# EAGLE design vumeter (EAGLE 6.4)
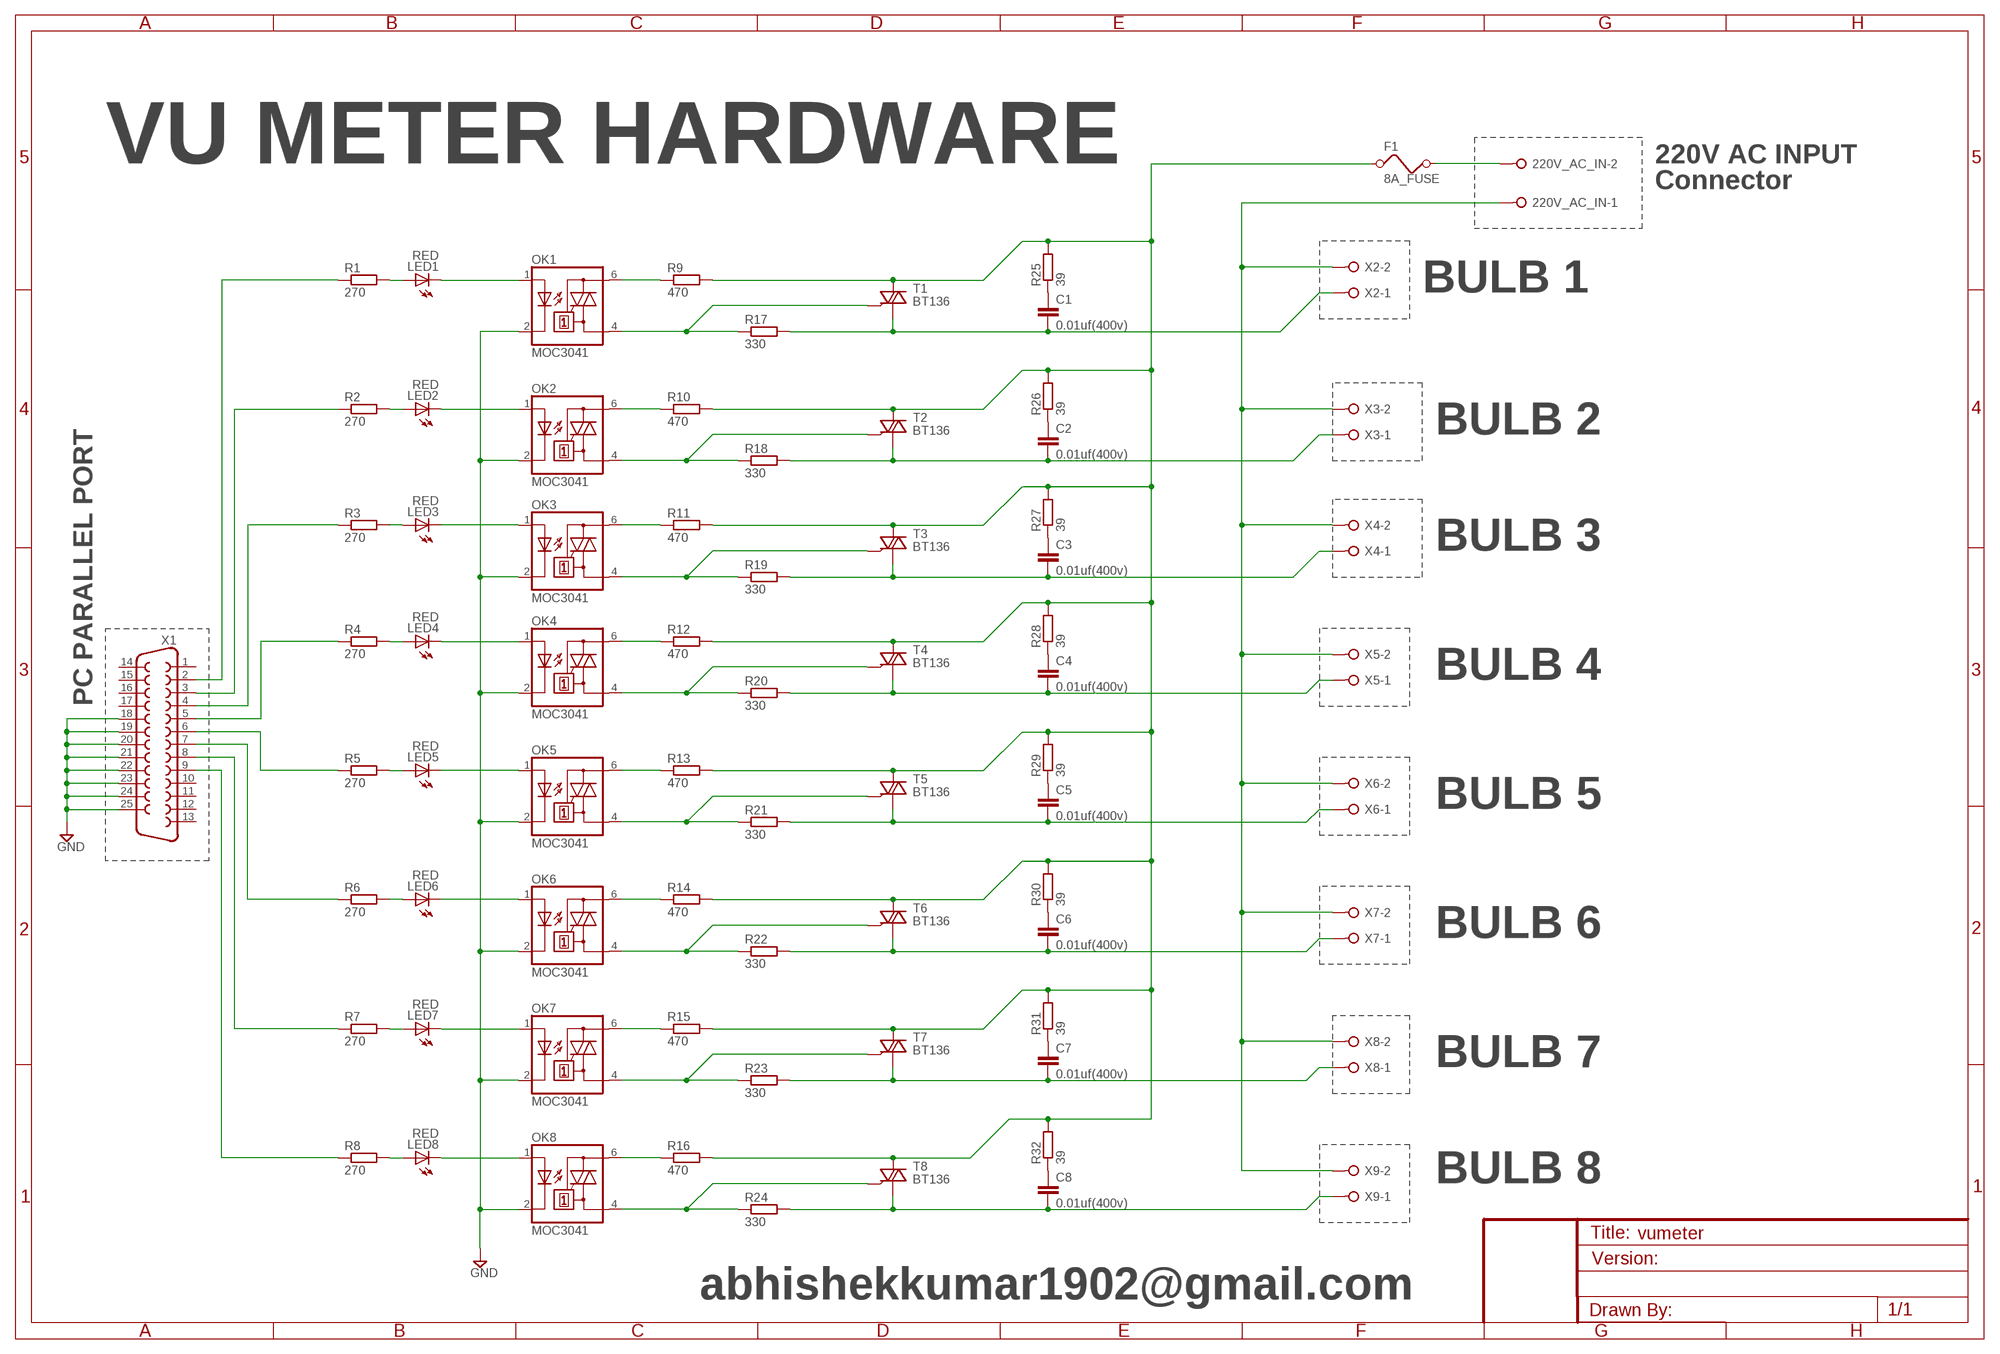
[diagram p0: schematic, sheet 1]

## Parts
220V_AC_IN  W237-02P  [W237-132]
C1  0.01uf(400v)  C-EU102-043X133  [C102-043X133]
C2  0.01uf(400v)  C-EU102-043X133  [C102-043X133]
C3  0.01uf(400v)  C-EU102-043X133  [C102-043X133]
C4  0.01uf(400v)  C-EU102-043X133  [C102-043X133]
C5  0.01uf(400v)  C-EU102-043X133  [C102-043X133]
C6  0.01uf(400v)  C-EU102-043X133  [C102-043X133]
C7  0.01uf(400v)  C-EU102-043X133  [C102-043X133]
C8  0.01uf(400v)  C-EU102-043X133  [C102-043X133]
F1  8A_FUSE  FUSE  [FUSE]
LED1  RED  LED3MM  [LED3MM]
LED2  RED  LED3MM  [LED3MM]
LED3  RED  LED3MM  [LED3MM]
LED4  RED  LED3MM  [LED3MM]
LED5  RED  LED3MM  [LED3MM]
LED6  RED  LED3MM  [LED3MM]
LED7  RED  LED3MM  [LED3MM]
LED8  RED  LED3MM  [LED3MM]
OK1  MOC3041  MOC3041T  [DIL06B]
OK2  MOC3041  MOC3041T  [DIL06B]
OK3  MOC3041  MOC3041T  [DIL06B]
OK4  MOC3041  MOC3041T  [DIL06B]
OK5  MOC3041  MOC3041T  [DIL06B]
OK6  MOC3041  MOC3041T  [DIL06B]
OK7  MOC3041  MOC3041T  [DIL06B]
OK8  MOC3041  MOC3041T  [DIL06B]
R1  270  R-EU_0309/12  [0309/12]
R2  270  R-EU_0309/12  [0309/12]
R3  270  R-EU_0309/12  [0309/12]
R4  270  R-EU_0309/12  [0309/12]
R5  270  R-EU_0309/12  [0309/12]
R6  270  R-EU_0309/12  [0309/12]
R7  270  R-EU_0309/12  [0309/12]
R8  270  R-EU_0309/12  [0309/12]
R9  470  R-EU_0309/12  [0309/12]
R10  470  R-EU_0309/12  [0309/12]
R11  470  R-EU_0309/12  [0309/12]
R12  470  R-EU_0309/12  [0309/12]
R13  470  R-EU_0309/12  [0309/12]
R14  470  R-EU_0309/12  [0309/12]
R15  470  R-EU_0309/12  [0309/12]
R16  470  R-EU_0309/12  [0309/12]
R17  330  R-EU_0309/12  [0309/12]
R18  330  R-EU_0309/12  [0309/12]
R19  330  R-EU_0309/12  [0309/12]
R20  330  R-EU_0309/12  [0309/12]
R21  330  R-EU_0309/12  [0309/12]
R22  330  R-EU_0309/12  [0309/12]
R23  330  R-EU_0309/12  [0309/12]
R24  330  R-EU_0309/12  [0309/12]
R25  39  R-EU_0309/12  [0309/12]
R26  39  R-EU_0309/12  [0309/12]
R27  39  R-EU_0309/12  [0309/12]
R28  39  R-EU_0309/12  [0309/12]
R29  39  R-EU_0309/12  [0309/12]
R30  39  R-EU_0309/12  [0309/12]
R31  39  R-EU_0309/12  [0309/12]
R32  39  R-EU_0309/12  [0309/12]
T1  BT136  [TO220AB]
T2  BT136  [TO220AB]
T3  BT136  [TO220AB]
T4  BT136  [TO220AB]
T5  BT136  [TO220AB]
T6  BT136  [TO220AB]
T7  BT136  [TO220AB]
T8  BT136  [TO220AB]
X1  F25HP  [F25HP]
X2  W237-02P  [W237-132]
X3  W237-02P  [W237-132]
X4  W237-02P  [W237-132]
X5  W237-02P  [W237-132]
X6  W237-02P  [W237-132]
X7  W237-02P  [W237-132]
X8  W237-02P  [W237-132]
X9  W237-02P  [W237-132]

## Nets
GND: OK1.2(C) OK2.2(C) OK3.2(C) OK4.2(C) OK5.2(C) OK6.2(C) OK7.2(C) OK8.2(C) X1.18 X1.19 X1.20 X1.21 X1.22 X1.23 X1.24 X1.25
N$1: LED5.A R5.2
N$2: LED1.A R1.2
N$3: LED1.K(C) OK1.1(A)
N$4: LED2.A R2.2
N$5: LED2.K(C) OK2.1(A)
N$6: LED3.K(C) OK3.1(A)
N$7: LED3.A R3.2
N$8: LED4.K(C) OK4.1(A)
N$9: LED4.A R4.2
N$10: LED6.A R6.2
N$11: LED7.A R7.2
N$12: LED8.A R8.2
N$13: LED8.K(C) OK8.1(A)
N$14: LED7.K(C) OK7.1(A)
N$15: LED6.K(C) OK6.1(A)
N$16: LED5.K(C) OK5.1(A)
N$17: R1.1 X1.2
N$18: R2.1 X1.3
N$19: R3.1 X1.4
N$20: R4.1 X1.5
N$21: R5.1 X1.6
N$22: R6.1 X1.7
N$23: R7.1 X1.8
N$24: R8.1 X1.9
N$25: 220V_AC_IN.1 X2.2 X3.2 X4.2 X5.2 X6.2 X7.2 X8.2 X9.2
N$26: OK5.6(A2) R13.1
N$27: OK6.6(A2) R14.1
N$28: OK7.6(A2) R15.1
N$29: OK8.6(A2) R16.1
N$30: OK4.6(A2) R12.1
N$31: OK3.6(A2) R11.1
N$32: OK2.6(A2) R10.1
N$33: OK1.6(A2) R9.1
N$34: OK1.4(A1) R17.1 T1.3(G)
N$35: OK2.4(A1) R18.1 T2.3(G)
N$36: OK3.4(A1) R19.1 T3.3(G)
N$37: OK4.4(A1) R20.1 T4.3(G)
N$38: OK5.4(A1) R21.1 T5.3(G)
N$39: OK6.4(A1) R22.1 T6.3(G)
N$40: OK7.4(A1) R23.1 T7.3(G)
N$41: OK8.4(A1) R24.1 T8.3(G)
N$42: C1.1 R25.1
N$43: C2.1 R26.1
N$44: C3.1 R27.1
N$45: C4.1 R28.1
N$46: C5.1 R29.1
N$47: C6.1 R30.1
N$48: C7.1 R31.1
N$49: C8.1 R32.1
N$50: F1.1 R9.2 R10.2 R11.2 R12.2 R13.2 R14.2 R15.2 R16.2 R25.2 R26.2 R27.2 R28.2 R29.2 R30.2 R31.2 R32.2 T1.2(A2) T2.2(A2) T3.2(A2) T4.2(A2) T5.2(A2) T6.2(A2) T7.2(A2) T8.2(A2)
N$51: C1.2 R17.2 T1.1(A1) X2.1
N$52: C7.2 R23.2 T7.1(A1) X8.1
N$59: C2.2 R18.2 T2.1(A1) X3.1
N$60: C3.2 R19.2 T3.1(A1) X4.1
N$61: C6.2 R22.2 T6.1(A1) X7.1
N$62: C5.2 R21.2 T5.1(A1) X6.1
N$63: C4.2 R20.2 T4.1(A1) X5.1
N$65: C8.2 R24.2 T8.1(A1) X9.1
N$66: 220V_AC_IN.2 F1.2
Unconnected: X1.1 X1.10 X1.11 X1.12 X1.13 X1.14 X1.15 X1.16 X1.17

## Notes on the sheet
- VU METER HARDWARE | 220V AC INPUT
- Connector
- BULB 1
- BULB 2
- BULB 3
- BULB 4
- PC PARALLEL PORT
- BULB 5
- BULB 6
- BULB 7
- BULB 8
- abhishekkumar1902@gmail.com

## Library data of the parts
220V_AC_IN X2-X9 = con-wago-508:W237-02P: WAGO SREW CLAMP; OC_FARNELL: unknown; OC_NEWARK: unknown
C1-C8 = resistor:C-EU: CAPACITOR, European symbol
F1 = special:FUSE: FUSE
LED1-LED8 = led:LED: LED
OK1-OK8 = optocoupler:MOC30*: 6-Pin DIP Zero-Cross Optoisolators Triac Driver Output (250/400 Volt Peak) Source: http://www.fairchildsemi.com/ds/MO/MOC3043-M.pdf; OC_FARNELL: unknown; OC_NEWARK: unknown
R1-R32 = resistor:R-EU_: RESISTOR, European symbol
T1-T8 = triac:BT136: Triac BT136 series E sensitive gate Source: http://www.nxp.com/acrobat_download/datasheets/BT136_SERIES_E_2.pdf
X1 = SparkFun:F25: D-SUB 25 25 Pin male connector. PCB edge mount for regular PCB thicknesses. This connector will connect directly to the back of a PC parallel port or through a normal DB25 extension cable (M/F). SKU: PRT-08287

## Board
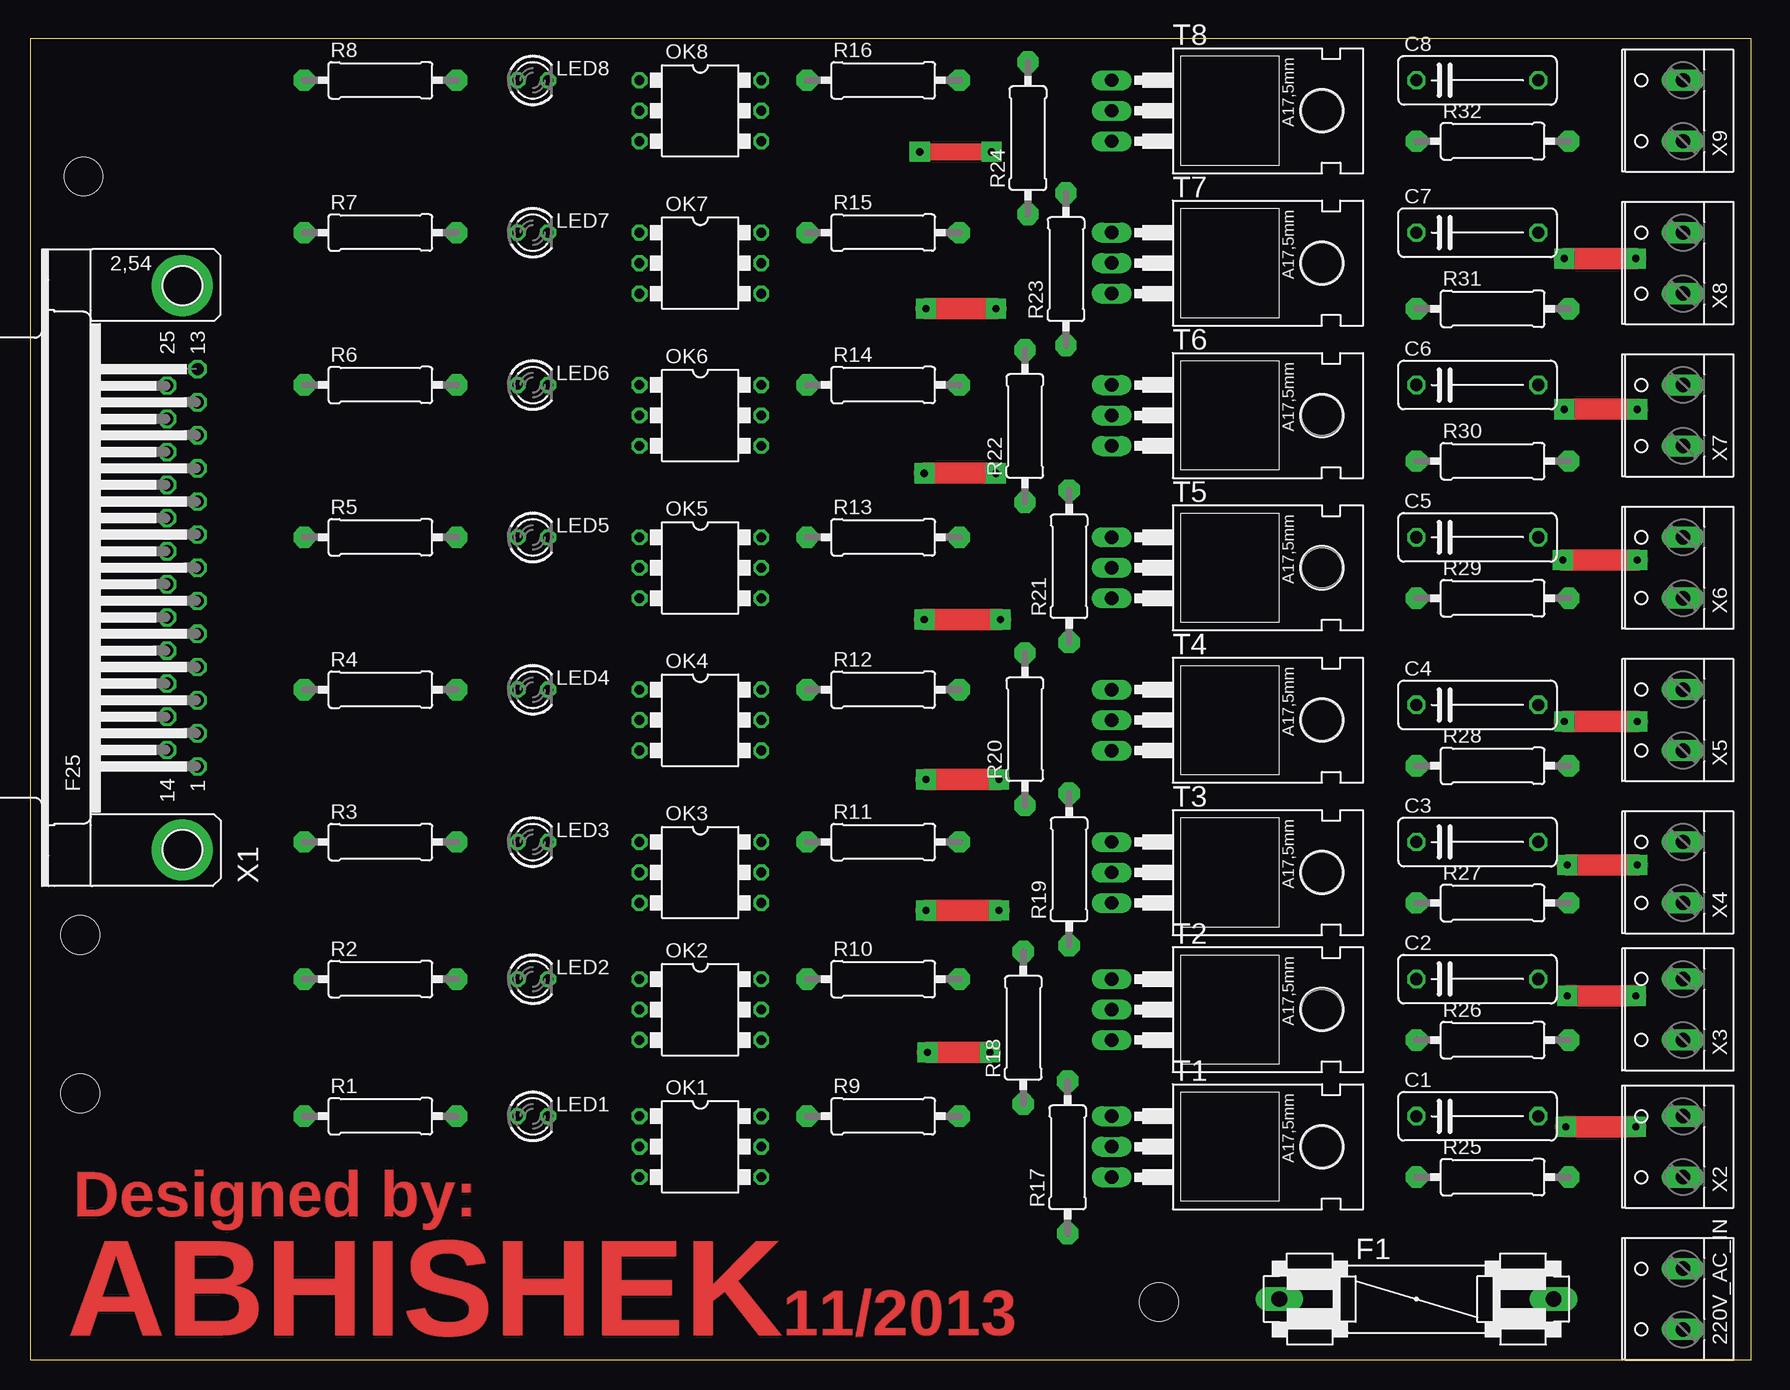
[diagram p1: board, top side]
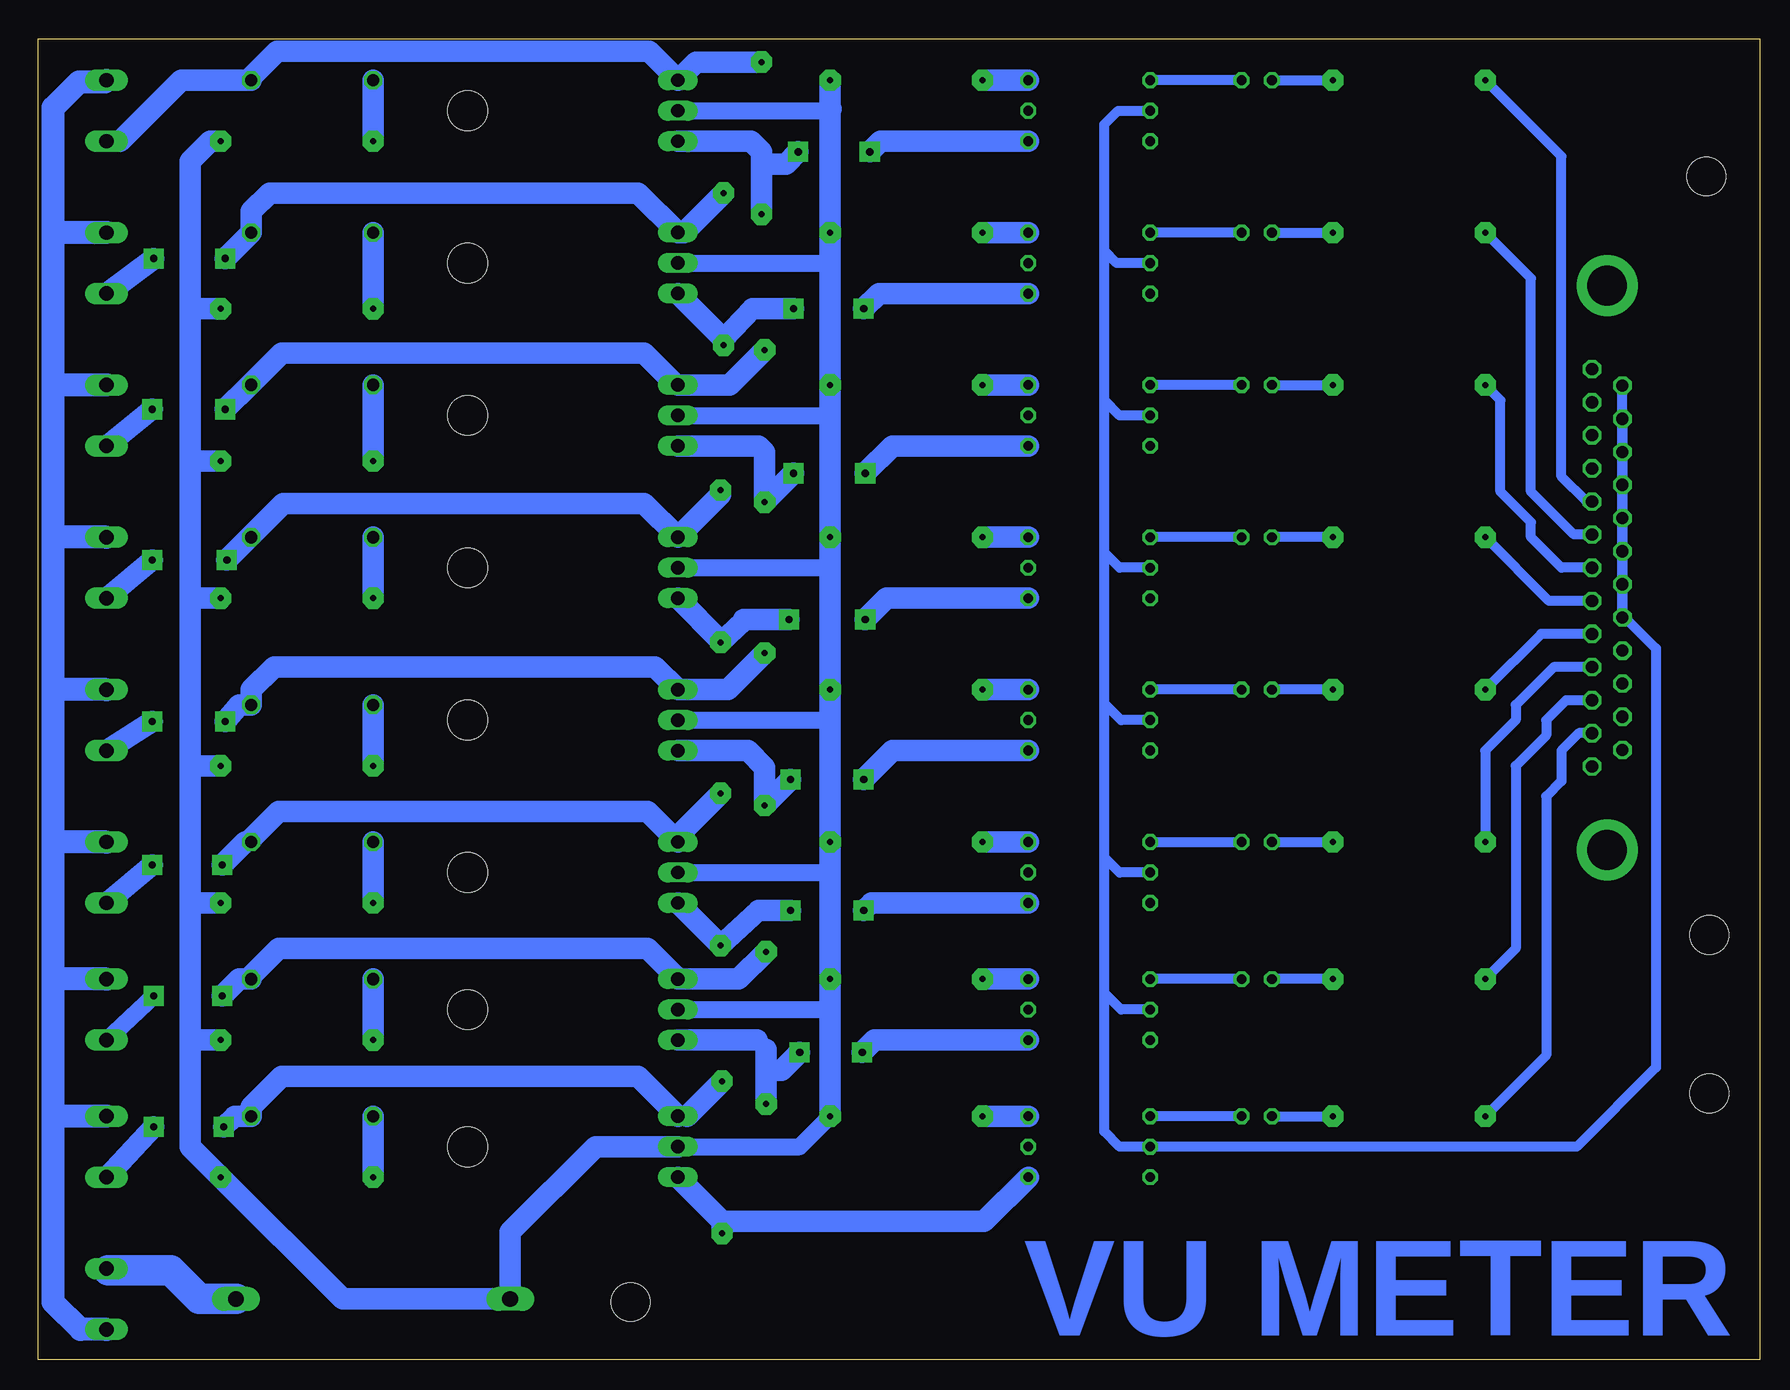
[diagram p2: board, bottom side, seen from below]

Size 143.49 x 110.16 mm. Coordinates in mm from the lower left corner, seen from the top.
Outline: 0,0 143.49,0 143.49,110.16 0,110.16 0,0
Copper layers (1*16): Top 0.035mm / dielectric 1.5mm / Bottom 0.035mm
Design rules "default": minimum track width 10mil, minimum drill 24mil, track to track 8mil, track to pad 8mil, pad to pad 8mil, via to via 8mil, smd to smd 8mil, copper to edge 40mil, drill to drill 8mil, minimum pad ring 10mil, minimum via ring 8mil, stop-mask expansion 4mil, vias tented up to drill 0mil, thermal gap 10mil
Holes 3.2 mm at 4.45,98.68 4.19,35.43 94.11,4.83 4.19,22.23

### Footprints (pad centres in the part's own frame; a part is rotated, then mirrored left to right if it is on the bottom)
W237-132 = drill 1.194 long: 1 -2.54,-0.635; 2 2.54,-0.635
C102-043X133 = drill 1.016 octagon: 1 -5.08,0; 2 5.08,0
FUSE = drill 1.321 long: 1 -11.43,0; 2 11.43,0
LED3MM = drill 0.813 octagon: A -1.27,0; K 1.27,0
DIL06B = drill 0.813 octagon: 1 -2.54,-5.08; 2 0,-5.08; 3 2.54,-5.08; 4 2.54,5.08; 5 0,5.08; 6 -2.54,5.08
0309/12 = drill 0.5 pad 1.778 octagon: 1 -6.35,0; 2 6.35,0
TO220AB = drill 1.118 long: 1 -2.54,-6.35; 2 0,-6.35; 3 2.54,-6.35 | hole 3.302: 0,11.176
F25HP = drill 1.016 octagon: 1 -16.561,-1.27; 2 -13.792,-1.27; 3 -11.049,-1.27; 4 -8.28,-1.27; 5 -5.512,-1.27; 6 -2.769,-1.27; 7 0,-1.27; 8 2.769,-1.27; 9 5.512,-1.27; 10 8.28,-1.27; 11 11.049,-1.27; 12 13.792,-1.27; 13 16.561,-1.27; 14 -15.189,1.27; 15 -12.421,1.27; 16 -9.652,1.27; 17 -6.909,1.27; 18 -4.14,1.27; 19 -1.372,1.27; 20 1.372,1.27; 21 4.14,1.27; 22 6.909,1.27; 23 9.652,1.27; 24 12.421,1.27; 25 15.189,1.27 | drill 3.302 pad 5.08: G1 -23.52,0; G2 23.52,0

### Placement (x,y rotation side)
220V_AC_IN  137.16,5.08 90 top
C1  120.65,20.32 0 top
C2  120.65,31.75 0 top
C3  120.65,43.18 0 top
C4  120.65,54.61 0 top
C5  120.65,68.58 0 top
C6  120.65,81.28 0 top
C7  120.65,93.98 0 top
C8  120.65,106.68 0 top
F1  115.57,5.08 0 top
LED1  41.91,20.32 0 top
LED2  41.91,31.75 0 top
LED3  41.91,43.18 0 top
LED4  41.91,55.88 0 top
LED5  41.91,68.58 0 top
LED6  41.91,81.28 0 top
LED7  41.91,93.98 0 top
LED8  41.91,106.68 0 top
OK1  55.88,17.78 270 top
OK2  55.88,29.21 270 top
OK3  55.88,40.64 270 top
OK4  55.88,53.34 270 top
OK5  55.88,66.04 270 top
OK6  55.88,78.74 270 top
OK7  55.88,91.44 270 top
OK8  55.88,104.14 270 top
R1  29.21,20.32 0 top
R2  29.21,31.75 0 top
R3  29.21,43.18 0 top
R4  29.21,55.88 0 top
R5  29.21,68.58 0 top
R6  29.21,81.28 0 top
R7  29.21,93.98 0 top
R8  29.21,106.68 0 top
R9  71.12,20.32 0 top
R10  71.12,31.75 0 top
R11  71.12,43.18 0 top
R12  71.12,55.88 0 top
R13  71.12,68.58 0 top
R14  71.12,81.28 0 top
R15  71.12,93.98 0 top
R16  71.12,106.68 0 top
R17  86.49,16.89 90 top
R18  82.8,27.69 90 top
R19  86.61,40.89 90 top
R20  82.93,52.58 90 top
R21  86.61,66.17 90 top
R22  82.93,77.85 90 top
R23  86.36,90.93 90 top
R24  83.19,101.85 90 top
R25  121.92,15.24 0 top
R26  121.92,26.67 0 top
R27  121.92,38.1 0 top
R28  121.92,49.53 0 top
R29  121.92,63.5 0 top
R30  121.92,74.93 0 top
R31  121.92,87.63 0 top
R32  121.92,101.6 0 top
T1  96.52,17.78 270 top
T2  96.52,29.21 270 top
T3  96.52,40.64 270 top
T4  96.52,53.34 270 top
T5  96.52,66.04 270 top
T6  96.52,78.74 270 top
T7  96.52,91.44 270 top
T8  96.52,104.14 270 top
X1  12.7,66.04 90 top
X2  137.16,17.78 90 top
X3  137.16,29.21 90 top
X4  137.16,40.64 90 top
X5  137.16,53.34 90 top
X6  137.16,66.04 90 top
X7  137.16,78.74 90 top
X8  137.16,91.44 90 top
X9  137.16,104.14 90 top

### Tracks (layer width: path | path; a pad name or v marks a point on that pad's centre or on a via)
GND
  Bottom 0.813: X1.18 X1.19 X1.20 X1.21 X1.22 X1.23 X1.24 | X1.24 X1.25 | 54.61,30.61 54.61,19.05 53.34,17.78 OK1.2 15.24,17.78 8.64,24.38 8.64,59.31 11.43,62.1 X1.24 | 54.61,30.61 54.61,41.91 | 54.61,41.91 54.61,54.74 | 54.61,54.74 54.61,67.31 | 54.61,67.31 54.61,80.01 | 54.61,80.01 54.61,92.46 | 54.61,92.46 54.61,103 53.47,104.14 OK8.2 | OK7.2 53.59,91.44 54.61,92.46 | OK6.2 53.34,78.74 54.61,80.01 | OK5.2 53.34,66.04 54.61,67.31 | OK4.2 53.21,53.34 54.61,54.74 | OK3.2 53.34,40.64 54.61,41.91 | OK2.2 53.21,29.21 54.61,30.61
N$1
  Bottom 0.813: R5.2 LED5.A
N$2
  Bottom 0.813: LED1.A R1.2
N$3
  Bottom 0.813: LED1.K OK1.1
N$4
  Bottom 0.813: R2.2 LED2.A
N$5
  Bottom 0.813: LED2.K OK2.1
N$6
  Bottom 0.813: OK3.1 LED3.K
N$7
  Bottom 0.813: LED3.A R3.2
N$8
  Bottom 0.813: LED4.K OK4.1
N$9
  Bottom 0.813: R4.2 LED4.A
N$10
  Bottom 0.813: LED6.A R6.2
N$11
  Bottom 0.813: LED7.A R7.2
N$12
  Bottom 0.813: LED8.A R8.2
N$13
  Bottom 0.813: LED8.K OK8.1
N$14
  Bottom 0.813: LED7.K OK7.1
N$15
  Bottom 0.813: LED6.K OK6.1
N$16
  Bottom 0.813: LED5.K OK5.1
N$17
  Bottom 0.813: X1.2 15.06,52.25 16.51,50.8 16.51,48.26 17.78,46.99 17.78,25.4 R1.1
N$18
  Bottom 0.813: X1.3 16.13,54.99 17.78,53.34 17.78,52.07 20.32,49.53 20.32,34.29 R2.1
N$19
  Bottom 0.813: X1.4 17.17,57.76 20.32,54.61 20.32,53.34 22.86,50.8 R3.1
N$20
  Bottom 0.813: X1.5 18.21,60.53 R4.1
N$21
  Bottom 0.813: X1.6 17.55,63.27 R5.1
N$22
  Bottom 0.813: X1.7 16.51,66.04 19.05,68.58 19.05,69.85 21.59,72.39 21.59,80.01 R6.1
N$23
  Bottom 0.813: X1.8 15.47,68.81 19.05,72.39 19.05,90.17 R7.1
N$24
  Bottom 0.813: X1.9 14.4,71.55 16.51,73.66 16.51,100.33 R8.1
N$25
  Bottom 1.27: 142.11,93.98 142.24,93.85 | 141.99,68.58 142.24,68.33 | 141.86,55.88 142.24,55.5 | 142.11,31.75 142.24,31.62 | 141.99,20.32 142.24,20.57
  Bottom 1.93: 220V_AC_IN.1 139.95,2.54 142.24,4.83 142.24,20.57 142.24,31.62 142.24,43.18 | 142.24,43.18 142.24,55.5 142.24,68.33 142.24,81.28 | 142.24,81.28 142.24,93.85 142.24,104.39 140.08,106.55 137.92,106.55 X9.2 | X8.2 142.11,93.98 | X7.2 142.24,81.28 | X6.2 141.99,68.58 | X5.2 141.86,55.88 | X4.2 142.24,43.18 | X3.2 142.11,31.75 | X2.2 141.99,20.32
N$26
  Bottom 1.778: OK5.6 R13.1
N$27
  Bottom 1.778: OK6.6 R14.1
N$28
  Bottom 1.778: OK7.6 R15.1
N$29
  Bottom 1.778: OK8.6 R16.1
N$30
  Bottom 1.778: OK4.6 R12.1
N$31
  Bottom 1.778: OK3.6 R11.1
N$32
  Bottom 1.778: OK2.6 R10.1
N$33
  Bottom 1.778: OK1.6 R9.1
N$34
  Bottom 1.778: R17.1 86.49,11.56 | 86.49,11.56 T1.3 | 86.49,11.56 64.64,11.56 OK1.4
N$35  (via drill 0.6 pad 1.68)
  Top 1.778: v74.8,25.65 v80.01,25.65
  Bottom 1.27: 83.57,26.67 82.8,25.91
  Bottom 1.422: 82.68,24.13 82.8,24
  Bottom 1.778: T2.3 83.57,26.67 | 82.8,25.91 82.8,24 R18.1 | OK2.4 73.79,26.67 v74.8,25.65 | v80.01,25.65 81.53,24.13 82.68,24.13
N$36  (via drill 0.6 pad 1.68)
  Top 1.778: v74.68,37.47 v80.77,37.47
  Bottom 1.778: T3.3 R19.1 83.44,37.47 v80.77,37.47 | OK3.4 74.04,38.1 v74.68,37.47
N$37  (via drill 0.6 pad 1.68)
  Top 1.778: v74.68,48.39 v80.77,48.39
  Bottom 1.778: T4.3 84.33,50.8 82.93,49.4 R20.1 v80.77,48.39 | OK4.4 72.26,50.8 v74.68,48.39
N$38  (via drill 0.6 pad 1.68)
  Top 1.778: v74.55,61.72 v80.9,61.72
  Bottom 1.27: R21.1 86.61,59.94
  Bottom 1.422: 84.71,61.72 84.71,61.59
  Bottom 1.778: 86.61,59.94 T5.3 | OK5.4 72.77,63.5 v74.55,61.72 | v80.9,61.72 84.71,61.72 | 84.71,61.59 R21.1
N$39  (via drill 0.6 pad 1.68)
  Top 1.778: v74.55,73.91 v80.52,73.91
  Bottom 1.778: T6.3 83.44,76.2 82.93,75.69 R22.1 v80.52,73.91 | OK6.4 72.26,76.2 v74.55,73.91
N$40  (via drill 0.6 pad 1.68)
  Top 1.778: v74.68,87.63 v80.52,87.63
  Bottom 1.27: R23.1 86.36,85.09
  Bottom 1.778: T7.3 86.36,85.09 83.95,87.63 v80.52,87.63 | OK7.4 73.41,88.9 v74.68,87.63
N$41  (via drill 0.6 pad 1.68)
  Top 1.422: v74.17,100.71 v80.14,100.71
  Bottom 1.778: T8.3 84.07,101.6 83.19,100.71 83.19,99.69 | 83.19,99.69 R24.1 | OK8.4 73.28,101.6 v74.17,100.71 | v80.14,100.71 81.15,99.69 83.19,99.69
N$42
  Bottom 1.778: R25.1 C1.1
N$43
  Bottom 1.778: R26.1 C2.1
N$44
  Bottom 1.778: R27.1 C3.1
N$45
  Bottom 1.778: R28.1 C4.1
N$46
  Bottom 1.778: R29.1 C5.1
N$47
  Bottom 1.778: R30.1 C6.1
N$48
  Bottom 1.778: R31.1 C7.1
N$49
  Bottom 1.778: R32.1 C8.1
N$50
  Bottom 1.27: 130.56,38.1 130.81,38.35 | 130.56,49.53 130.81,49.78 | 130.68,74.93 130.81,74.8 | 130.56,87.63 130.81,87.38
  Bottom 1.422: T8.2 77.6,104.14 | T1.2 80.01,17.78 R9.2 | T2.2 77.47,29.21 | T3.2 77.72,40.64 | T4.2 77.6,53.34 77.47,53.47 | T5.2 77.72,66.04 77.47,65.79 | T6.2 77.85,78.74 77.47,79.12 | T7.2 77.72,91.44 77.47,91.19
  Bottom 1.778: R32.2 129.16,101.6 130.81,99.95 130.81,87.38 130.81,74.8 130.81,63.5 | 130.81,63.5 130.81,49.78 130.81,38.35 130.81,26.67 | 130.81,26.67 130.81,17.78 R25.2 118.11,5.08 F1.1 104.14,10.67 97.03,17.78 T1.2 | R26.2 130.81,26.67 | R27.2 130.56,38.1 | R28.2 130.56,49.53 | R29.2 130.81,63.5 | R30.2 130.68,74.93 | R31.2 130.56,87.63 | R9.2 77.47,29.21 R10.2 77.47,40.89 | 77.47,40.89 R11.2 77.47,53.47 R12.2 77.47,65.79 R13.2 77.47,79.12 R14.2 77.47,91.19 R15.2 77.47,104.27 R16.2 | 77.72,40.64 77.47,40.89
  Bottom 1.93: 77.6,104.14 77.47,104.27
N$51  (via drill 0.6 pad 1.68)
  Top 1.778: v128.02,19.43 v133.86,19.43
  Bottom 1.27: T1.1 89.41,20.32
  Bottom 1.778: T1.1 93.47,23.62 123.19,23.62 125.73,21.08 C1.2 127.13,20.32 v128.02,19.43 | 89.41,20.32 R17.2 | v133.86,19.43 X2.1
N$52  (via drill 0.6 pad 1.68)
  Top 1.778: v127.89,91.82 v133.86,91.82
  Bottom 1.778: R23.2 89.66,93.98 T7.1 93.47,97.28 124.21,97.28 125.73,95.76 C7.2 v127.89,91.82 | v133.86,91.82 X8.1
N$59  (via drill 0.6 pad 1.68)
  Top 1.778: v128.14,30.35 v133.86,30.35
  Bottom 1.27: C2.2 125.73,32
  Bottom 1.422: v133.86,30.35 X3.1
  Bottom 1.778: 125.73,32 123.44,34.29 92.71,34.29 T2.1 85.09,31.75 R18.2 | C2.2 126.75,31.75 v128.14,30.35
N$60  (via drill 0.6 pad 1.68)
  Top 1.778: v128.14,41.27 v133.99,41.27
  Bottom 1.27: C3.2 125.73,43.43 | T3.1 90.17,43.69
  Bottom 1.422: C3.2 126.24,43.18
  Bottom 1.778: 125.73,43.43 123.44,45.72 92.71,45.72 T3.1 | 90.17,43.69 R19.2 | 126.24,43.18 v128.14,41.27 | v133.99,41.27 X4.1
N$61  (via drill 0.6 pad 1.68)
  Top 1.778: v127.89,79.25 v133.99,79.25
  Bottom 1.27: C6.2 125.73,81.41 | 90.55,81.53 90.42,81.53 T6.1
  Bottom 1.422: C6.2 125.86,81.28
  Bottom 1.778: 125.73,81.41 123.19,83.95 92.96,83.95 90.55,81.53 | T6.1 85.85,81.28 R22.2 | 125.86,81.28 v127.89,79.25 | v133.99,79.25 X7.1
N$62  (via drill 0.6 pad 1.68)
  Top 1.778: v127.76,66.67 v133.99,66.67
  Bottom 1.27: C5.2 125.73,68.71 | R21.2 86.61,72.14
  Bottom 1.422: C5.2 125.86,68.58
  Bottom 1.778: 125.73,68.71 123.06,71.37 92.96,71.37 T5.1 86.61,72.14 | 125.86,68.58 v127.76,66.67 | v133.99,66.67 X6.1
N$63  (via drill 0.6 pad 1.68)
  Top 1.778: v127.89,53.21 v133.99,53.21
  Bottom 1.778: R20.2 85.98,55.88 T4.1 92.08,57.79 123.83,57.79 125.73,55.88 C4.2 126.75,54.61 v127.89,53.21 | v133.99,53.21 X5.1
N$65
  Bottom 1.27: C8.2 125.73,106.93
  Bottom 1.778: 125.73,106.93 123.57,109.09 92.58,109.09 T8.1 88.65,108.2 R24.2 | X9.1 136.65,101.6 131.57,106.68 C8.2
N$66
  Bottom 1.27: 137.67,7.49 220V_AC_IN.2
  Bottom 2.54: F1.2 130.05,5.08 132.46,7.49 137.67,7.49

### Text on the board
Top: Designed by: | ABHISHEK | 11/2013
Bottom: VU METER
